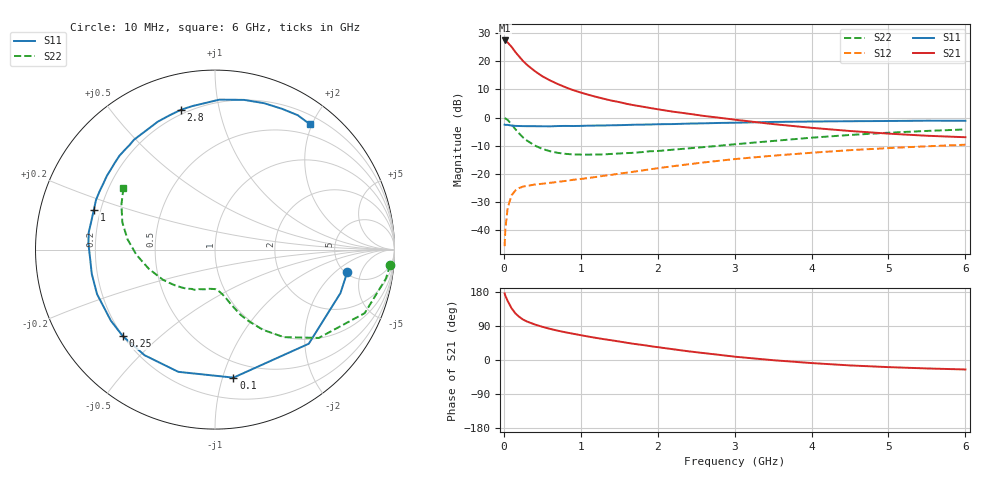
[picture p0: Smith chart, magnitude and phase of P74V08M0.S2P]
! SIEMENS Small Signal Semiconductors
! BFP196
! Si NPN RF Bipolar Junction Transistor in SOT143
! VCE = 4 V  IC = 8 mA
! Common Emitter S-Parameters:  May  1996
# GHz  S  MA  R  50
!  f  S11  S21  S12  S22
! GHz  MAG  ANG  MAG  ANG  MAG  ANG  MAG  ANG
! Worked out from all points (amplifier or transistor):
!   36 points, 10 MHz to 6 GHz, reference 50 ohm
!   highest |S21| = 27.4 dB at 10 MHz (marker M1)
!   |S21| within 3 dB of that: start of sweep to 120.4 MHz
!   unconditionally stable (mu >= 1): 958.1 MHz to 3.232 GHz
!   at 250 MHz: K = 0.34, MSG = 22.3 dB, |S12| = -24.5 dB
!   at 1.4 GHz: K = 1.14, MAG = 10.9 dB, |S12| = -20.3 dB
!   at 6 GHz: K = 0.97, MSG = 1.3 dB, |S12| = -9.7 dB
!   S11 on the Smith chart (normalised r, x): 10 MHz: 5.15, -2.97; 100 MHz: 0.37, -1.09; 250 MHz: 0.20, -0.38; 1 GHz: 0.17, +0.16; 2.8 GHz: 0.18, +0.77; 6 GHz: 0.33, +1.97
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0.01  0.7473 -9.8  23.38 175.7  0.0052 86.8  0.9795 -5.0
0.02  0.7399 -19.1  22.83 169.5  0.0104 79.2  0.966 -9.6
0.05  0.7403 -45.1  21.46 155.7  0.0251 68.4  0.9061 -23.0
0.1  0.7207 -81.8  18.06 136.7  0.0416 53.5  0.7592 -40.4
0.15  0.7111 -106.7  14.58 123.0  0.0506 43.0  0.6208 -51.8
0.2  0.7074 -123.7  12.08 113.8  0.0561 37.2  0.5201 -59.2
0.25  0.7045 -136.9  10.09 106.7  0.0594 33.8  0.4426 -64.6
0.3  0.7025 -145.7  8.662 101.6  0.0611 31.9  0.3906 -68.6
0.4  0.7024 -159.3  6.709 93.9  0.0645 29.8  0.3192 -73.6
0.5  0.6998 -168.8  5.411 87.6  0.0667 29.5  0.2777 -77.2
0.6  0.6979 -176.6  4.567 82.2  0.0694 30.4  0.2523 -80.6
0.7  0.7063 177.2  3.945 77.4  0.0718 31.6  0.2363 -83.8
0.8  0.71 172.1  3.456 73.2  0.0749 32.9  0.2268 -86.6
1  0.7106 161.8  2.779 65.5  0.081 35.4  0.2199 -91.3
1.1  0.7182 157.4  2.535 61.8  0.0845 36.5  0.2196 -94.3
1.6  0.7387 139.0  1.747 45.5  0.1053 40.9  0.2336 -109.0
2.2  0.7659 120.3  1.271 28.4  0.1368 41.6  0.2689 -125.8
2.8  0.8018 103.7  0.992 13.6  0.1711 38.3  0.3157 -144.2
3.5  0.8359 88.3  0.765 -0.5  0.2102 31.8  0.3839 -163.8
4.5  0.8604 71.4  0.577 -14.3  0.2634 20.9  0.4906 173.3
5.5  0.8792 58.4  0.475 -22.3  0.3088 9.2  0.5786 154.3
6  0.8761 52.9  0.447 -25.0  0.3291 2.9  0.6151 146.0
